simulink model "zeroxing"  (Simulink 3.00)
settings: Solver=VariableStepDiscrete  SolverMode=SingleTasking  StartTime=0.0  StopTime=10  RelTol=1e-3  AbsTol=1e-6

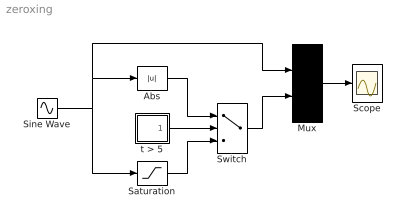
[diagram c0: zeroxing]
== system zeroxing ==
  Abs : Abs
  Mux : Mux  Inputs=2
  Saturation : Saturate  UpperLimit=[0.5 .55 .6]  LowerLimit=[-0.5 -.55 -.6]
  Scope : Scope
  Sine Wave : Sin  Amplitude=1  Frequency=1  Phase=[.1 .2 .3]  SampleTime=0
  Switch : Switch  Threshold=0.5
  t > 5 : Subsystem
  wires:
  t > 5/1(t > 5) -> Switch/2
  Switch/1 -> Mux/2
  Saturation/1 -> Switch/3
  Abs/1 -> Switch/1
  Sine Wave/1 -> Abs/1, Mux/1, Saturation/1
  Mux/1 -> Scope/1

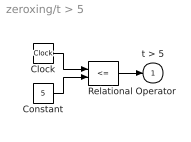
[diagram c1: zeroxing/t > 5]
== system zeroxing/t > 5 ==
  Clock : Clock
  Constant : Constant  Value=5
  Relational Operator : RelationalOperator  Operator=<=
  t > 5 : Outport  Port=1  InitialOutput=0
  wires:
  Constant/1 -> Relational Operator/2
  Clock/1 -> Relational Operator/1
  Relational Operator/1 -> t > 5/1
